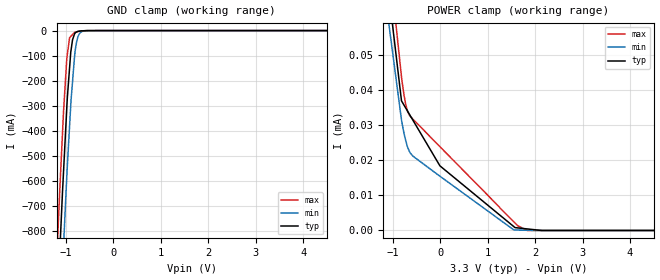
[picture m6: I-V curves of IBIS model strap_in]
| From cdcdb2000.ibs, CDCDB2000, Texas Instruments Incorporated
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[Model]   strap_in
Model_type   Input
Vinl = 0.9
Vinh = 2.4
|   typ   min   max
C_comp   0.857pF   0.829pF   0.863pF
[Voltage Range]   3.3   3.135   3.465
[Temperature Range]   27   105   -40
[Power Clamp Reference]   3.3   3.135   3.465
[GND Clamp Reference]   0   0   0
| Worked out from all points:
|   GND clamp passes 1 mA (typ) near -0.66 V on its own axis
|   POWER clamp passes 1 mA (typ) near -3.21 V on its own axis
[GND Clamp]
|   Voltage   I(typ)   I(min)   I(max)
-3.3V     -11.22A    -11.44A    -11.05A
-1.169V   -1.043A    -1.347A    -794.9mA
-1.117V   -822.5mA   -1.123A    -578.3mA
-1.052V   -561.2mA   -858mA     -321.1mA
-981.8mV  -301.2mA   -575.6mA   -108.9mA
-924.3mV  -147.1mA   -378.9mA   -28.1mA
-900.2mV  -86.51mA   -297.9mA   -23.31mA
-862.2mV  -36.61mA   -202.8mA   -15.76mA
-814.3mV  -11.45mA   -92.87mA   -6.235mA
-733.4mV  -2.541mA   -18mA      -3.463mA
-576.2mV  -221.8uA   -584.9uA   -329.7uA
6.6V      0A         0A         0A
[POWER Clamp]
|   Voltage   I(typ)   I(min)   I(max)
-3.3V     1.075mA    586.4uA    1.556mA
-1.562V   121.9uA    107.8uA    138.5uA
-818.7mV  36.87uA    31.43uA    43.75uA
-783.2mV  36.07uA    28.83uA    40.16uA
-734.9mV  34.96uA    25.9uA     36.22uA
-701mV    34.19uA    24.15uA    34.32uA
-623.1mV  32.41uA    21.86uA    32.33uA
-8.584mV  18.39uA    15.45uA    23.85uA
1.553V    1.069uA    134.7nA    2.429uA
1.833V    440.5nA    59.79nA    0A
2.136V    0A         0A         0A
6.6V      0A         0A         0A
